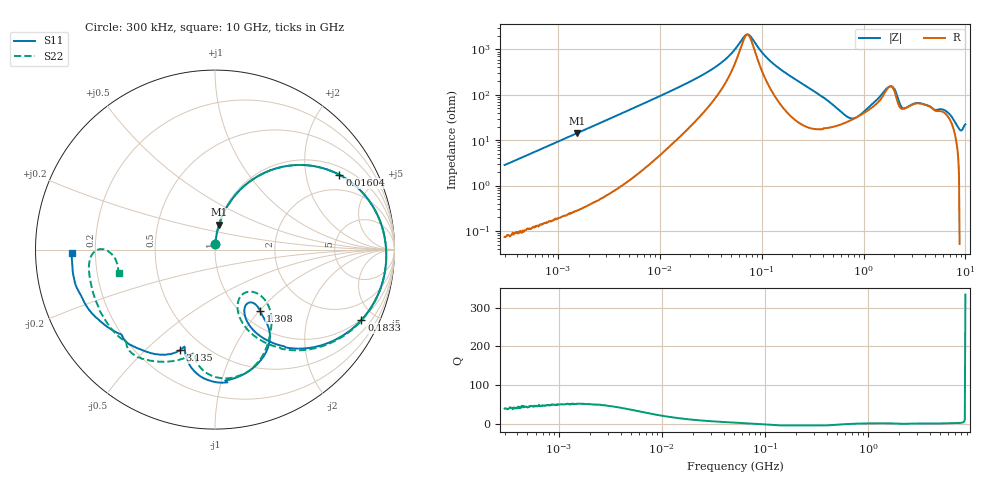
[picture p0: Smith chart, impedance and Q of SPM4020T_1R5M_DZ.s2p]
! S-Parameter Data Generated by TDK Corporation
! Copyright(C) 2024 TDK Corporation.
! All Rights Reserved.
! TDK P/N: SPM4020T-1R5M-DZ (SMD / SMT Inductor (Coil))
! Property: L=1.5uH at 100kHz
! Size(LxWxT): 4.3x4.1x2mm
! Model Type: s2p (Touchstone File Format Version 1.0)
! Frequency: DC=Yes Start=0.3MHz Stop=10000MHz 802points Log-sweep
! Model Generated on May 28, 2024
! Terms and conditions regarding TDK Simulation Models:
! 1)This simulation model is being provided solely for informational
!  purposes. Please refer to the specifications of the products in
!  terms of detailed characteristics of such products.
! 2)In no event shall TDK Corporation of any of its subsidiaries be
!  liable for any loss or damage arising, directly or indirectly,
!  from any information contained in this simulation model, including,
!  but not limited to loss or damages arising from any inaccuracies,
!  omissions or errors in connection with such information.
! 3)Any and all copyrights on this simulation model are owned by
!  TDK Corporation.  Duplication or redistribution of this simulation
!  model without prior written permission from TDK Corporation
!  is prohibited.
! 4)This simulation model is subject to any modification or change
!  without any prior notice.
! 5)Neither TDK Corporation nor any of its subsidiaries shall make any
!  warranty, express or implied, including but not limited to the
!  correctness, implied warranties of merchantability and fitness for
!  a particular purpose with respect to this simulation models.
! 6)The use of this simulation model shall be deemed to have consented
!  to the terms and conditions hereof.
! Port Assignments:
!  1 ---@@@--- 2
! Applicable Conditions:
!  Temperature = 25 degC
!  DC Bias Current = 0 A
!  Small Signal Operation
# Hz S MA R 50
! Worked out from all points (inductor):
!   801 points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, 300 kHz to 10 GHz, reference 50 ohm
!   read as one part in series: L = 1.49 uH near 318.3 kHz
!   highest Q = 51 at 1.55 MHz (marker M1), where L = 1.47 uH
!   self-resonance near 72.35 MHz
!   S11 on the Smith chart (normalised r, x): 300 kHz: 1.00, +0.06; 16.04 MHz: 1.29, +3.11; 183.3 MHz: 0.96, -4.17; 1.308 GHz: 1.21, -1.01; 3.135 GHz: 0.37, -0.64; 10 GHz: 0.11, -0.01
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300000  0.02871 87.2  0.9986 -1.6  0.9985 -1.6  0.0288 87.9
1550270  0.1411 80.7  0.9873 -8.2  0.9872 -8.1  0.1411 80.7
1713600  0.1555 79.9  0.9848 -9.0  0.9847 -9.0  0.1555 79.9
4363314  0.3688 66.7  0.92 -21.8  0.92 -21.8  0.3688 66.7
9671944  0.6533 46.2  0.7265 -41.1  0.7266 -41.1  0.6532 46.1
1.603896e7  0.8088 31.1  0.5269 -54.4  0.527 -54.4  0.8087 31.0
3.424315e7  0.9256 12.0  0.236 -66.5  0.236 -66.5  0.9256 11.9
5.477226e7  0.9502 2.6  0.09447 -58.2  0.09451 -58.2  0.9503 2.4
7.414452e7  0.9554 -3.3  0.04508 5.9  0.04511 5.9  0.9555 -3.6
1.161426e8  0.9473 -13.1  0.1538 61.0  0.1538 61.0  0.9473 -13.5
1.833272e8  0.9049 -25.7  0.3202 56.2  0.3202 56.2  0.9045 -26.4
3.126428e8  0.7706 -45.0  0.5461 36.9  0.5462 36.9  0.7674 -46.3
6.738867e8  0.4231 -65.9  0.7368 -5.5  0.7369 -5.5  0.3927 -70.0
9.560117e8  0.3501 -57.8  0.6956 -28.3  0.6956 -28.3  0.292 -56.9
1.307877e9  0.423 -53.5  0.5641 -50.4  0.5641 -50.4  0.3924 -45.2
1.767019e9  0.6667 -67.5  0.3214 -56.6  0.3214 -56.6  0.6104 -61.6
2.325038e9  0.66 -102.3  0.4449 -42.5  0.445 -42.5  0.6556 -97.7
3.135132e9  0.5936 -109.2  0.3835 -75.0  0.3835 -75.0  0.6336 -106.3
6.091595e9  0.7268 -141.9  0.2461 -116.0  0.2461 -116.0  0.7233 -138.2
7.987505e9  0.7866 -159.7  0.1718 -144.4  0.1719 -144.4  0.7172 -164.0
9.217363e9  0.8023 -170.1  0.1263 -157.8  0.1266 -157.8  0.661 -179.7
1e10  0.7995 -178.7  0.1053 -154.4  0.1055 -154.4  0.5537 -166.1
